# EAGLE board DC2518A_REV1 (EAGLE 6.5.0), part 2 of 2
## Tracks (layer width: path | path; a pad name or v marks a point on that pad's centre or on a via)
+2V5  (via drill 0.25)
  Top 0.152: v38.86,29.21 39.12,29.46 39.91,29.46 U9.13 U9.14
  Bottom 0.152: C41.1 v38.86,29.21
+3V3  (via drill 0.25)
  Top 0.152: U9.12 U9.11 38.59,30.5 v37.97,31.11 | v14.73,13.21 16.13,13.21 C15.1 16.22,13.21 17.02,13.21 17.45,12.78 U4.2 19.63,12.78 21.08,14.22 23.88,14.22 24.38,13.72 24.41,13.74 U3.6 | C50.1 84.07,18.76 84.07,19.56 84.29,19.77 U12.8 | 84.51,13.35 R80.R4_2 84.44,13.34 83.69,13.34 83.57,13.21 83.57,12.57 82.55,12.57 82.22,12.24 82.22,9.27 U11.18 | R66.2 v65.91,2.03 | SW1.SW1 15.29,29 15.62,29.46 25.27,29.46 v25.78,28.96 | R68.2 23.7,57.84 v24.38,57.28 | R69.2 53.34,56.9 53.85,56.39 v54.48,56.39 | v61.72,43.81 61.72,41.77 R58.2 | v69.09,45.97 69.48,46.37 R54.2 73.21,46.37 R53.2 C37.1
  Top 0.203: M10.2 94.68,35.21 C48.1 R72.1 R73.1 94.65,29.81 96.27,28.19 96.27,19.81 95.38,18.92 90,18.92 | R67.2 v22.99,2.03 | 90,19.43 90,18.92 | 90,18.92 R77.1 89.95,17.7 R81.1 | R80.R4_2 R80.R3_2 R80.R2_2 R80.R1_2 84.58,16.07 v84.58,17.02 84.58,17.27 84.16,17.69 C50.1 85.6,18.67 86.36,19.43 90,19.43 | v65.91,2.03 v77.22,2.03 | 90,19.43 90,20.45 R74.1 | R70.2 R71.1 25.95,29.12 v25.78,28.96
  Route2 0.152: v69.09,45.97 63.88,45.97 v61.72,43.81
  Route2 0.203: v14.73,2.03 v22.99,2.03 v44.45,2.03 v65.91,2.03 | v77.22,17.02 82.3,17.02 82.55,16.76 83.31,16.76 83.57,17.02 v84.58,17.02 | v37.97,31.11 v31.75,31.11 27.94,31.11 v25.78,28.96
  Route15 0.152: v54.48,56.39 58.04,56.39 61.72,52.7 v61.72,43.81 v61.72,32.38
  Route15 0.203: v14.73,2.03 v14.73,13.21 | v43.94,15.88 43.94,14.99 44.45,14.48 v44.45,2.03 | v77.22,2.03 v77.22,17.02 | v24.38,57.28 24.38,48.13 v31.75,40.01 v31.75,31.11 | v37.97,21.84 v37.97,31.11
  Bottom 0.152: 43.92,21.89 43.94,21.89 | 40.64,15.88 R16.1 | v25.78,28.96 25.78,27.9 R31.1 | C40.1 v37.97,31.11 | R36.2 31.24,40.51 v31.75,40.01 | R47.1 62.57,43.81 v61.72,43.81 | 42.56,22.35 R62.R1_2 42.61,21.84 v37.97,21.84 | 47.5,23.11 48.26,23.11 49.66,24.51 54.99,24.51 56.48,26 R65.2 R64.2 R63.2 56.48,32.38 58.93,32.38 | 47.5,23.11 46.99,23.11 45.85,21.89 R62.R4_2 | 58.93,32.38 v61.72,32.38 | v31.75,31.11 31.75,31.66 C45.1 30.48,32.51 28.96,32.51 28.32,33.15 U10.5 | 47.5,23.11 R14.1 47.79,22.19 47.88,22.1 49.02,22.1 49.66,21.59 50.29,21.59 50.55,21.34 M1.2 | R94.2 58.04,35.69 58.93,34.8 58.93,32.38
  Bottom 0.203: R62.R1_2 R62.R2_2 43.92,21.89 R62.R3_2 R62.R4_2 | 43.94,21.89 v43.94,15.88 40.64,15.88
+12V  (via drill 0.25)
  Top 0.152: 55.82,45.65 55.88,45.59 | 51.59,44.4 L2.1 | R93.2 R92.2 89.5,36.87 88.77,37.59 86.23,37.59 84.58,39.24 TP14.TP1
  Top 0.203: U7.3 55.82,45.65 | 55.88,45.59 55.88,44.7
  Top 0.229: 55.88,44.7 55.88,44.55 arc-90 55.73,44.4 55.63,44.4
  Top 0.254: 55.63,44.4 51.59,44.4
  Top 0.305: v48.26,45.72 v47.24,45.72 | v52.07,45.72 v52.96,45.72 v51.05,45.72 v50.16,45.72
  Bottom 0.305: C58.2 78.74,25.4 79.12,25.78 80.57,25.78 U14.20 80.64,29.59 81.53,30.48 81.92,30.48 81.92,31.53 U14.3
  other vias: 38.1,43.43 38.1,44.2 38.99,43.43 38.99,44.2
  pour Bottom (no thermals): 89.66,42.67 89.66,41.66 87.38,41.66 86.61,40.64 86.61,33.15 82.8,33.15 82.07,32.49 82.07,30.86 81.81,30.86 81.81,32.99 82.3,33.53 86.11,33.53 86.11,37.85 81.28,37.85 80.77,38.35 80.77,40.77 80.01,41.53 77.47,41.53 77.47,39.88 75.69,39.88 75.18,41.02 66.17,41.02 66.17,39.62 65.79,39.62 65.79,41.02 36.96,41.02 36.96,44.45 37.47,44.83 37.47,46.23 53.59,46.23 53.59,45.47 56.13,43.43 80.77,43.43 82.04,44.7 84.84,44.7 86.36,42.67
  pour Bottom (no thermals): 77.6,24.89 80.77,24.89 80.77,29.59 81.53,30.35 82.07,30.35 82.07,30.86 81.79,30.86 81.79,30.61 81.53,30.61 77.6,26.8
  pour Top (no thermals): 47.24,45.72 48.26,45.72 48.26,44.45 47.24,44.45
  pour Top (no thermals): 50.16,45.72 52.96,45.72 52.96,44.45 50.16,44.45
+12V_IN  (via drill 0.25)
  Top 0.152: v37.97,33.02 37.97,31.88 38.86,31 U9.10 | v98.04,43.18 98.72,42.51 R78.1 R83.2
  Route2 0.305: v92.71,39.12 89.15,35.56 v37.97,35.56
  Route15 0.305: v37.97,35.56 v37.97,33.02
  Route15 0.813: JP2.13 JP2.14
  Bottom 0.152: C39.1 v37.97,33.02 | v98.04,43.18 96.31,43.18 96.06,42.93
  Bottom 0.305: 93.98,42.16 93.98,39.12 v92.71,39.12
  Bottom 0.813: C52.2 96.01,45.09 96.01,48.47 J1.1 96.06,42.93 96.06,42.21 96.01,42.16 93.98,42.16 92.14,42.16 R84.I1
  pour Bottom (no thermals): 92.46,59.31 93.85,59.31 94.36,58.8 94.36,52.2 95.38,51.18 97.03,51.18 98.68,49.53 98.68,44.96 98.04,44.32 97.54,44.32 96.77,43.43 96.77,31.11 94.36,28.57 94.36,10.16 94.11,9.91 94.11,3.56 93.73,3.17 92.71,3.17 92.46,3.43 92.46,21.72 93.6,22.86 93.6,28.32 93.47,28.45 93.47,54.86 92.46,55.88
+15V  (via drill 0.25)
  other vias: 62.61,21.21 63.93,18.62 63.93,17.73 64.64,19.81
  pour Bottom (no thermals): 72.39,29.72 72.39,39.37 72.64,39.88 74.68,39.88 74.68,28.83 74.17,28.19 73.15,28.19 73.15,21.08 73.53,20.7 76.07,20.7 76.71,21.34 81.79,21.34 82.5,21.77 82.5,24.21 81.79,24.89 81.79,26.29 82.04,26.29 82.04,25.02 82.68,24.38 82.68,21.59 81.41,20.32 73.53,20.32 73.15,19.94 73.15,15.24 72.64,14.73 62.23,14.73 60.71,16.26 60.71,22.61 61.98,23.88 67.06,23.88
  pour Top (no thermals): 65.02,19.05 65.02,19.94 64.64,20.32 64.14,20.32 64.14,21.59 62.23,21.59 61.34,22.48 59.56,22.48 59.56,20.95 61.72,20.95 63.5,19.18 63.5,17.91 62.1,17.91 62.1,15.75 63.5,15.75 63.88,16.13 63.88,16.89 64.39,17.4 64.39,18.41
-15V  (via drill 0.25)
  Top 0.152: R19.2 26.38,12.41 26.67,12.7 28.07,12.7 28.07,13.46 | U3.1 25.91,16.99 25.91,15.7 | 28.07,15.7 U3.PAD
  Top 0.254: U4.4 18.09,11.12 18.16,11.05 v18.92,11.05
  Top 0.305: 25.91,15.7 28.07,15.7
  Top 0.406: U3.3 U3.2 U3.1 25.92,19.55 24.77,20.95 C11.1
  Route2 0.152: v89.15,18.49 88.9,18.29 v76.2,18.29
  Route15 0.152: v90.81,33.78 90.81,29.97 89.15,28.32 v89.15,18.49
  Bottom 0.152: R91.1 v89.15,18.49 | v76.2,18.29 76.17,18.32 D4.A
  Bottom 0.254: C14.1 v18.92,11.05
  other vias: 27.56,13.46 28.57,13.46 27.56,17.27 28.57,17.27
  pour Bottom (no thermals): 73.91,19.43 75.69,19.43 75.69,13.46 72.77,10.54 25.4,10.41 17.27,10.41 17.27,11.56 24,11.56 24,16 25.53,17.78 28.83,17.78 29.34,17.27 36.83,17.27 40.01,14.1 73.03,14.1 73.91,14.99 73.91,19.18 74.04,19.3
  pour Top (no thermals): 27.3,17.4 28.83,17.4 28.83,13.34 27.3,13.34
A0_MUX  (via drill 0.25)
  Top 0.152: U11.3 85.34,5.84 84.84,5.33 81.92,5.33 80.52,6.73 80.52,8.94 80.72,9.22 v80.7,9.65 80.7,10.03 80.52,10.21 80.52,10.67 80.64,10.79 80.64,14.48 81.28,15.11 82.57,15.11 R80.R2_1
  Bottom 0.152: JP3.6 81.79,8.64 80.77,9.65 v80.7,9.65
A1_MUX  (via drill 0.25)
  Top 0.152: U11.2 84.84,6.1 84.45,5.71 82.04,5.71 80.9,6.86 80.9,8.89 81.28,9.27 81.28,9.91 81.15,10.03 v81.15,10.41 81.15,10.79 81.03,10.92 81.03,11.43 81.15,11.56 81.15,13.84 81.66,14.35 82.57,14.35 R80.R3_1
  Bottom 0.152: JP3.7 81.79,9.91 81.28,10.41 v81.15,10.41
A2_MUX  (via drill 0.25)
  Top 0.152: U11.1 84.34,6.37 84.07,6.1 82.17,6.1 81.28,6.99 81.28,8.76 81.66,9.14 81.66,9.91 81.79,10.03 81.79,10.67 81.66,10.79 v81.66,11.18 81.66,13.34 81.79,13.46 82.57,13.46 R80.R4_1 82.49,13.34
  Bottom 0.152: JP3.8 v81.66,11.18
ALERTB  (via drill 0.25)
  Top 0.152: v47.75,24.13 47.75,25.78 47.88,25.91 47.88,26.16 | 47.88,26.16 47.88,26.42 47.7,26.59 U9.31 | v54.86,26.92 54.1,26.16 47.88,26.16
  Route2 0.152: v12.32,24.13 12.95,24.13 13.21,23.88 30.1,23.88 30.35,24.13 46.23,24.13 46.35,24.21 46.86,24.21 46.99,24.13 v47.75,24.13 | v54.86,26.92 v69.09,26.92 | v71.37,5.21 81.84,5.21 JP2.3 | v25.78,30.48 v12.32,30.48
  Route15 0.152: JP2.3 83.25,4.63 82.68,5.21 81.28,5.21 79.76,6.73 79.76,10.92 80.01,11.18 80.01,54.86 80.26,55.12 82.8,55.12 83.31,55.63 83.31,56.59 JP1.3 | v12.32,24.13 v12.32,30.48 12.32,33.53 TP10.TP | v69.09,26.92 69.09,7.49 v71.37,5.21
  Bottom 0.152: U10.1 28.97,31 28.45,30.48 v25.78,30.48 | R65.1 54.78,28.28 54.86,28.19 v54.86,26.92
CTRL  (via drill 0.25)
  Top 0.152: R82.2 90.68,30.99 92.71,28.96 S1.2 S1.5 92.71,20.61 C51.1 | U9.32 48.26,27.3 49.02,27.3 | U9.22 | U9.22 U9.23 | U9.33 49.02,27.93 49.02,27.3 | U9.22 43.2,26.57 42.93,26.29 v42.16,26.29 | 49.02,27.3 v49.91,27.3
  Route2 0.152: v49.91,27.3 54.36,27.3 54.61,27.56 68.71,27.56 69.09,27.94 v78.23,27.94 86.23,27.94 86.36,28.07 87.12,28.07 87.25,27.94 91.69,27.94 S1.2
  Route15 0.152: JP1.2 80.49,58.64 78.49,56.64 78.49,38.61 77.85,37.97 77.85,37.08 78.23,36.7 v78.23,27.94 78.23,5.84 80.01,4.06 80.01,3.03 JP2.2 | v42.16,26.29 42.16,25.78 42.93,25.02 43.69,25.02 44.2,25.53 44.2,26.04 45.47,27.3 v49.91,27.3
  Bottom 0.152: R64.1 53.59,30.86 53.59,27.3 v49.91,27.3
CTRL_P  (via drill 0.25)
  Top 0.152: R82.1 88.39,31.2 88.39,31.88 v89.03,32.51
  Route15 0.152: v89.03,32.51 89.28,32.77 TP8.TP
EESCL  (via drill 0.25)
  Route2 0.152: v102.5,12.97 102,12.97 101.35,12.32 v96.14,12.32
  Route15 0.152: J2.11 v102.5,12.97
  Bottom 0.152: R76.1 96.14,13.42 v96.14,12.32 95.25,12.32 95.25,10.54 96.27,9.78 96.27,8 95.57,7.56 U13.1
EESDA  (via drill 0.25)
  Route2 0.152: J2.12 104.5,21.83 99.57,16.89 96.39,16.89 v96.14,16.64
  Bottom 0.152: v96.14,16.64 96.14,15.53 R75.1 95.38,15.49 94.74,14.86 94.74,10.41 95.38,9.9 U13.3
FAULTB  (via drill 0.25)
  Top 0.152: 44.7,26.67 U9.25 U9.26 44.78,27.25 44.7,27.18 44.7,26.67 | 44.7,26.67 v44.7,25.27
  Route2 0.152: v13.21,25.4 24,25.4 24.51,24.89 29.84,24.89 30.1,25.15 43.18,25.15 43.31,25.02 43.81,25.02 44.07,25.27 v44.7,25.27 | v43.69,1.4 77.98,1.4 77.98,3.81 81.23,3.81 JP2.1 | v25.78,31.5 v13.21,31.5
  Route15 0.152: JP1.1 79.77,56.66 78.99,55.88 78.87,37.97 79.12,37.72 79.12,37.21 78.87,36.96 78.87,6.18 JP2.1 | TP9.TP 13.21,41.53 v13.21,31.5 v13.21,25.4 | v44.7,25.27 43.18,23.75 43.18,14.61 43.69,14.1 v43.69,1.4
  Bottom 0.152: U10.3 25.82,31.54 v25.78,31.5 | R62.R2_1 43.54,24.64 43.57,24.64 44.2,25.27 v44.7,25.27
GND  (via drill 0.25)
  Top 0.203: Q3.1 20.59,43.7 20.57,42.67 Q3.3
  other vias: 85.85,53.34 82.04,40.64 82.93,17.4 57.15,46.48 57.15,45.47 43.94,32.26 44.96,32.26 43.94,31.24 44.96,31.24
  pour Bottom (rank 2, no thermals): 0.51,0.51 0.51,62.99 106.17,62.99 106.17,0.51
  pour Top (rank 3): 0.51,0.51 106.17,0.51 106.17,62.99 0.51,62.99
  pour Route2 (no thermals): 0.51,0.51 106.17,0.51 106.17,62.99 0.51,62.99
  pour Route15 (no thermals): 0.51,0.51 106.17,0.51 106.17,62.99 0.51,62.99
  pour Route15: 86.61,55.63 86.87,55.63 86.87,53.85 86.36,53.34 86.36,50.29 86.87,49.78 86.87,44.7 86.61,44.45 86.61,43.94 86.87,43.69 86.87,16.51 86.61,16.26 86.36,16.51 86.36,21.59 86.61,21.84 86.61,22.35 86.36,22.61 85.34,22.61 85.09,22.23 85.09,21.72 85.34,21.34 85.34,12.7 86.11,11.94 86.11,7.11 85.34,6.35 83.31,6.35 82.55,7.11 82.55,8.64 82.8,8.89 82.8,12.7 81.53,13.97 81.53,24.64 82.8,24.64 82.8,23.88 85.6,23.88 85.85,24.13 85.85,24.64 85.34,25.15 84.58,25.15 84.07,25.65 81.53,25.65 81.53,46.74 85.09,50.29 85.09,53.59 86.36,54.86 86.61,54.86
  pour Top: 53.49,33.73 54.2,33.73 54.2,33.71 53.49,33.71
  pour Top: 52.76,34.11 52.78,34.11 52.78,33.45 52.76,33.45
  pour Bottom: 14.02,49.11 14.68,49.11 14.68,49.07 14.02,49.07
IIN_SNSM  (via drill 0.25)
  Top 0.152: v44.7,38.1 44.7,37.72 44.58,37.6 44.58,37.08 44.7,36.96 44.7,36.93 U9.56
  Route2 0.152: v88.65,39.12 87.76,38.23 55.24,38.23 54.99,37.97 52.96,37.97 52.83,38.1 v44.7,38.1
  Bottom 0.152: R84.E2 88.65,40.3 v88.65,39.12
IIN_SNSP  (via drill 0.25)
  Top 0.152: v45.21,37.34 45.2,37.33 U9.55 | U9.9 39.24,31.5 v38.86,31.88
  Route2 0.152: v91.44,39.12 91.44,38.73 88.65,36.07 65.79,36.07 65.02,36.78 64.26,36.78 64.14,36.7 49.28,36.7 49.15,36.78 48.9,36.78 48.77,36.7 45.85,36.7 v45.21,37.34 43.05,37.34 42.42,37.97 40.01,37.97 39.88,37.9 39.62,37.9 39.5,37.97 v38.86,37.97
  Route15 0.152: v38.86,31.88 v38.86,37.97
  Bottom 0.152: R84.E1 91.95,40.2 91.95,39.37 91.69,39.12 v91.44,39.12
ISNSN_CH0  (via drill 0.25)
  Top 0.152: U9.42 51.84,32.51 52.01,32.42 52.46,32.42 52.58,32.51 v53.85,32.51 U$40.P$2 | v72.01,8 R8.2 72.06,9.13 | R1.2 v68.33,15.88
  Route2 0.152: v54.61,8 v68.33,8 v72.01,8
  Route15 0.152: v53.85,32.51 53.85,9.02 v54.61,8 | v68.33,15.88 v68.33,8
ISNSN_CH1  (via drill 0.25)
  Top 0.152: v19.3,18.67 R20.2 21.46,18.76 | U9.44 48.95,33.53 49.53,33.53 49.66,33.45 50.16,33.45 50.29,33.53 v51.56,33.53 51.82,33.78 U$39.P$2 | R24.2 v19.3,9.14
  Route2 0.152: v51.56,19.05 47.24,19.05 46.99,19.3 19.94,19.3 v19.3,18.67
  Route15 0.152: v51.56,33.53 51.56,32.38 51.69,32.26 51.69,31.62 51.56,31.5 v51.56,19.05 | v19.3,9.14 19.3,10.41 19.56,10.67 19.56,11.43 19.3,11.68 v19.3,18.67
ISNSN_CH2  (via drill 0.25)
  Top 0.152: v51.05,34.54 50.29,34.54 50.16,34.67 49.66,34.67 49.53,34.54 48.99,34.54 U9.46
  Route2 0.152: v13.97,34.54 15.75,34.54 15.88,34.67 16.38,34.67 16.51,34.54 27.05,34.54 27.18,34.42 27.69,34.42 27.81,34.54 28.83,34.54 28.96,34.42 29.46,34.42 29.59,34.54 36.83,34.54 36.96,34.47 37.47,34.47 37.59,34.54 49.53,34.54 49.66,34.67 50.16,34.67 50.29,34.54 v51.05,34.54
  Route15 0.152: v14.48,43.81 13.97,43.31 v13.97,34.54
  Bottom 0.152: U$41.P$2 14.35,47.28 R39.2 14.39,45.01 C24.2 14.44,43.85 v14.48,43.81
ISNSN_CH3  (via drill 0.25)
  Top 0.152: U9.48 49.02,35.57 v49.02,36.2 | v72.39,43.56 72.77,43.56 72.9,43.69 R53.1 C37.2 76.33,44.87 TP30.1
  Route2 0.152: v49.02,36.2 v64.64,36.2 | v72.39,43.56 68.33,43.56 68.2,43.69 67.18,43.69 67.06,43.56 v65.79,43.56
  Route15 0.152: v64.64,36.2 65.79,37.34 v65.79,43.56
  Bottom 0.152: v65.79,43.56 M5.3
ISNSP_CH0  (via drill 0.25)
  Top 0.152: U9.41 49.65,32 49.78,32.08 50.04,32.08 50.16,32 50.93,32 v51.05,31.95 | v48.51,21.21 48.51,19.39 C7.1 R11.1 R12.1 48.3,14.48
  Route15 0.152: v51.05,31.95 51.05,27.18 48.77,24.89 48.77,21.59 v48.51,21.21 47.12,21.21 46.1,20.19 TP27.1
ISNSP_CH1  (via drill 0.25)
  Top 0.152: R25.1 R26.1 | U9.43 51.21,33.02 51.33,32.92 51.8,32.92 51.89,33.02 v52.2,33.02 | v41.91,16.64 41.4,16.64 41.02,16.26 R26.1 | C16.1 40.27,16.69 R26.1
  Route2 0.152: v51.56,16.64 v41.91,16.64
  Route15 0.152: v52.2,33.02 52.2,17.27 v51.56,16.64 | TP28.1 42.67,16 v41.91,16.64
ISNSP_CH2  (via drill 0.25)
  Top 0.152: v49.91,34.04 48.99,34.04 U9.45
  Route2 0.152: v16.13,34.04 27.05,34.04 27.18,33.91 27.69,33.91 27.81,34.04 28.83,34.04 28.96,33.91 29.46,33.91 29.59,34.04 v49.91,34.04 | TP29.1 16.13,54.86 v16.13,48.77
  Route15 0.152: v16.13,48.77 v16.13,34.04
  Bottom 0.152: U6.1 16.13,50.97 v16.13,48.77 16.13,47.28 R39.1 16.09,45.01 C24.1
ISNSP_CH3  (via drill 0.25)
  Top 0.152: U9.47 50.11,35 50.29,35.18 51.31,35.18 v51.94,34.54 | v70.36,44.2 R54.1
  Route2 0.152: v51.94,34.54 v70.61,34.54 | 72.14,44.2 v70.36,44.2
  Route15 0.152: v70.61,34.54 70.61,35.05 70.36,35.31 v70.36,44.2
N$1  (via drill 0.25)
  Top 0.152: v47.24,37.34 47.2,37.29 U9.51
  Bottom 0.152: v47.24,37.34 47.71,37.76 47.71,38.35 C43.1
N$2
  Top 0.152: R43.2 R42.1
N$3  (via drill 0.25)
  Top 0.152: v56.13,8.64 55.37,8.64 54.74,9.27 54.74,10.16 55.12,10.54 R6.1 | 62.48,18.5 U1.16 62.57,18.41 60.2,18.41 v60.2,19.3 | R5.2 53.12,18.2 53.34,18.41 57.04,18.41 U1.1 | R7.1 69.83,9.18 v70.61,9.17
  Top 0.203: v72.01,19.3 72.1,19.22 C6.1 72.1,16.42 72.39,16.13 72.39,15.28 U2.5
  Route2 0.152: v56.13,8.64 70.61,8.64 v70.61,9.17
  Route2 0.203: v72.01,19.3 64.9,19.3 64.77,19.18 64.01,19.18 63.88,19.3 v60.2,19.3
  Bottom 0.152: D7.A 59.69,18.8 v60.2,19.3
  pour Top (no thermals): 55.37,9.27 58.42,9.27 58.8,9.65 60.45,9.65 60.45,12.19 61.98,13.72 62.99,13.72 62.99,13.97 61.47,13.97 61.47,17.91 61.85,18.29 62.99,18.29 62.99,18.54 56.64,18.54 56.64,15.62 58.17,15.62 58.17,13.97 56.64,13.97 56.64,13.72 58.42,13.72 58.42,12.7 57.66,11.81 55.37,11.81
N$4
  Top 0.152: LED7.A 92.85,40.52 92.96,40.64 R83.1
N$5
  Top 0.152: U1.6 56.09,15.15 55.75,15.49 55.75,17.53 R5.1
N$6
  Top 0.152: U1.11 63.92,15.15 64.39,15.62 64.39,16.38 64.9,16.89 65.41,16.89 65.41,17.87 R2.1
N$7  (via drill 0.25)
  Top 0.152: R12.2 50.8,14.61 v51.18,14.48 | U1.10 62.61,14.48 v65.53,14.48 65.53,15.79 R1.1 65.41,15.84
  Route2 0.152: v51.18,14.48 v65.53,14.48
N$8  (via drill 0.25)
  Top 0.152: U2.4 72.52,13.27 72.52,12.45 73.53,11.43 73.53,6.73 61.59,6.73 TP3.TP | v54.74,12.19 54.74,10.92 54.36,10.54 R6.2 | R10.P$2 56.39,20.7 v56.39,19.81
  Route15 0.152: v56.39,19.81 54.74,18.54 v54.74,12.19
  pour Top (no thermals): 52.58,11.81 54.1,11.81 54.1,7.62 55.63,6.1 60.2,6.1 60.96,5.33 60.96,4.32 60.2,3.56 55.63,3.56 54.48,2.41 51.31,2.41 51.31,4.06 51.69,4.45 51.69,5.21 51.31,5.59 51.31,8 52.58,9.27
N$9
  Bottom 0.152: R38.1 17.4,50.2 17.4,52.83 16.15,52.83
  Bottom 0.203: 16.15,52.83 U6.3
N$10  (via drill 0.25)
  Top 0.152: U2.1 69.92,15.19 70.87,15.19 71.37,14.68 71.37,12.7 72.01,11.94 R8.1 71.34,10.92 v70.74,10.92 | R11.2 49.28,16.76 v49.28,10.29
  Route2 0.152: v49.28,10.29 70.36,10.29 v70.74,10.92
N$11
  Top 0.152: U3.8 29.21,14.39 29.21,18.54 29.84,19.05 30.73,19.05 | 30.73,19.05 30.7,19.81 R17.2 | C10.2 30.73,19.05
N$12  (via drill 0.25)
  Top 0.152: R18.2 34.04,19.81 34.04,21.55 R17.1 32.77,21.72 32,21.72 v30.99,22.86
  Bottom 0.152: v30.99,22.86 30.1,22.86 29.72,23.24 Q5.3
N$13  (via drill 0.25)
  Top 0.152: R21.1 v33.66,11.94 | v23.19,15.11 23.19,16.34 R22.1
  Route2 0.152: v33.66,11.94 v23.29,11.94
  Route15 0.152: v23.29,11.94 23.29,14.81 v23.19,15.11
  pour Top (no thermals): 33.66,17.27 29.72,17.27 29.72,15.62 31.62,15.62 32.38,14.86 32.38,12.57 34.92,12.57 34.92,13.84 33.66,15.11
N$14  (via drill 0.25)
  Route15 0.152: v30.99,18.54 29.46,17.02 29.46,9.14 v29.21,8.89
  Bottom 0.152: R28.2 30.99,19.3 v30.99,18.54 | v29.21,8.89 TP4.TP
  pour Top (no thermals): 29.97,12.06 29.97,6.86 29.21,6.1 28.83,6.1 27.94,5.21 27.94,4.32 28.7,3.56 32,3.56 32.77,2.79 35.69,2.79 35.69,5.71 35.43,5.97 35.43,8.38 34.92,8.89 34.92,11.05 30.73,11.05 30.73,12.06
N$15
  Top 0.152: U4.1 19.52,13.43 21.5,15.41 R22.2
N$16  (via drill 0.25)
  Top 0.152: R81.2 91.69,14.57 v91.69,13.59
  Bottom 0.152: v91.69,13.59 91.82,13.46 91.82,7.37 JP3.4
N$17  (via drill 0.25)
  Top 0.152: R26.2 37.47,16.26 v37.47,15.24 | U3.5 24.77,14.39 v24.77,15.24 24.77,17.78 24.13,18.54 23.24,18.54 23.24,18.63 R20.1
  Route2 0.152: v37.47,15.24 v24.77,15.24
N$18
  Top 0.152: U4.8 23.4,13.43 23.88,12.95 23.88,10.79 24.13,10.54 28.45,10.54 28.7,10.79 28.7,11.6 R23.2
N$19  (via drill 0.25)
  Top 0.152: R25.2 38.48,13.97 v38.48,10.16 | R24.1 22.06,9.99 22.35,10.29 | 22.35,10.29 22.35,11.42 U4.5 | 22.35,10.29 22.73,10.29 v23.11,10.16
  Route2 0.152: v38.48,10.16 v23.11,10.16
N$20
  Top 0.152: R35.2 R40.1 27.43,45.51 U5.3
  Top 0.203: R35.2 R34.1
N$21
  Bottom 0.152: Q5.2 30.67,29.72 24.13,29.72 24.13,27.81 R31.2 R32.2
N$22
  Top 0.254: U5.5 31.11,46.48 31.88,45.21 C20.1
N$23  (via drill 0.25)
  Top 0.152: C21.1 22.09,49.4 | v21.08,53.21 25.27,53.21 25.53,52.96 R37.1
  Bottom 0.152: R38.2 v21.08,53.21 | 18.67,50.99 18.67,51.82 21.08,51.82
  Bottom 0.203: U6.5 18.67,50.99 | 21.08,51.82 R38.2 C23.1
  pour Top (no thermals): 20.7,48.51 24.13,48.51 24.38,48.77 25.65,48.77 25.65,50.04 26.8,50.93 26.8,52.58 24.26,52.58 24.26,50.8 23.5,50.04 20.7,50.04
N$24  (via drill 0.25)
  Top 0.152: R50.2 71.48,52.25 71.48,52.76 71.27,52.93 69.55,52.93 69.47,52.91 69.34,52.83 R49.1 69.34,51.31 v71.37,51.31
  Bottom 0.152: v71.37,51.31 70.36,51.31 | 70.36,51.31 69.09,51.31 68.58,51.82 68.58,53.34 67.82,54.1 67.82,54.78 C35.2 | 70.36,49.4 70.36,48.51 69.98,48.16 69.22,48.16 68.58,48.77 U8.2 | 70.36,49.4 72.09,49.4 D5.A | 70.36,49.4 70.36,51.31
  pour Top (no thermals): 61.85,49.15 63.25,49.15 63.25,50.42 63.88,51.05 70.61,51.05 70.61,52.53 61.85,52.53
N$25
  Top 0.152: R66.1 64.1,5.8 63.88,5.59 LED1.A
N$26
  pour Top (no thermals): 26.8,47.12 28.07,47.12 28.07,48.01 28.57,48.51 28.83,48.51 29.46,49.15 29.46,50.04 30.48,50.8 30.48,53.98 29.08,53.98 29.08,51.31 27.69,49.91 27.69,48.77 26.8,48.13
N$27
  Top 0.152: U3.4 26.87,15.04 26.92,14.99 26.92,13.46 26.42,12.95 24.89,12.95 24.64,12.7 24.64,11.72 R19.1
N$28  (via drill 0.25)
  Top 0.152: R51.2 74.8,53.14 71.78,53.14 71.65,53.26 69.7,53.26 69.34,53.59 R49.2 | v66.78,50.34 66.64,50.13 R52.2 66.8,49.11 | v65.53,56.39 59.69,56.39 TP6.TP | R55.2 67.69,41.67 v67.69,42.6
  Route15 0.152: v65.53,56.39 65.53,51.56 v66.78,50.34 67.69,49.43 v67.69,42.6 67.69,37.34 67.06,36.7 v66.67,36.7
  Bottom 0.152: v66.67,36.7 66.29,36.21 R95.1
  pour Top (no thermals): 70.61,54.1 70.61,55.63 71.88,56.9 74.68,56.9 74.68,58.17 67.06,58.17 66.04,59.18 60.96,59.18 60.2,59.94 59.18,59.94 58.42,59.18 58.42,58.17 59.18,57.4 66.29,57.4 68.07,55.63 68.07,54.1
N$29  (via drill 0.25)
  Top 0.152: v37.85,53.47 40.64,53.47 40.77,53.43 R42.2 | R37.2 25.53,53.72 25.4,53.59 23.5,53.59 22.99,54.1 v20.19,54.1 | R34.2 21.59,41.06 v21.59,41.02
  Route2 0.152: v37.85,53.47 32.51,58.67 TP5.TP
  Route15 0.152: v21.59,41.02 20.19,41.02 v20.19,54.1
  Bottom 0.152: U6.4 20.13,52.89 20.19,52.96 v20.19,54.1
  pour Top (no thermals): 24.26,54.1 26.8,54.1 26.8,54.74 27.43,55.12 39.62,55.12 39.88,55.24 39.88,57.02 31.88,57.02 30.48,58.17 30.48,59.18 29.72,59.94 28.7,59.94 27.94,59.18 27.94,57.53 24.26,55.5
N$30  (via drill 0.25)
  Top 0.152: SW1.SW2 21.29,26.72 v22.99,24.77
  Route2 0.152: v22.99,24.77 23.5,24.77 23.88,24.38 29.97,24.38 30.23,24.64 46.99,24.64 47.12,24.77 56.01,24.77 56.39,25.15 v57.28,25.15
  Bottom 0.152: M2.1 59.69,23 59.69,23.5 59.09,24.09 R13.2 58.17,25.02 58.04,25.15 v57.28,25.15
N$31
  Top 0.152: U7.6 59.24,45.59 58.42,45.59 58.42,43.56 56.52,43.56 55.5,42.55 R45.1
N$32  (via drill 0.25)
  other vias: 34.29,47.12 35.05,47.12 35.05,47.88 34.29,47.88 34.29,48.64 35.05,48.64
  pour Top (no thermals): 29.46,47.62 29.46,47.12 31.24,47.12 31.75,46.61 35.43,46.61 35.43,54.1 31.5,54.1 31.5,50.8 33.78,50.8 33.78,48.13 31.62,48.13 31.11,47.62
  pour Bottom (no thermals): 37.08,45.72 37.08,46.99 35.69,48.26 35.69,49.28 33.78,49.28 33.78,46.74 34.8,45.72
N$33  (via drill 0.25)
  Top 0.152: v60.83,46.35 60.78,46.3 U7.7
  Bottom 0.152: C31.1 60.87,46.39 v60.83,46.35
N$34
  Bottom 0.152: R46.2 59.56,48.9 59.82,49.15 60.74,49.15 C32.1
N$35  (via drill 0.25)
  Top 0.152: U7.2 55.7,46.3 55.88,46.48 v55.88,48.77
  Bottom 0.152: R46.1 56.52,48.9 56.39,48.77 v55.88,48.77 55.63,48.51 55.63,44.45 C33.1
N$36  (via drill 0.25)
  Top 0.152: v54.99,47.62 U7.1 | R52.1 64.94,48.3 v64.9,48.26 | R59.1 57.26,42.56 v57.15,42.67
  Route2 0.152: v64.9,48.26 64.01,47.62 v54.99,47.62
  Route15 0.152: v57.15,42.67 56.01,42.67 54.99,43.69 v54.99,47.62
N$37  (via drill 0.25)
  Bottom 0.254: 51.44,49.02 v51.82,49.02 51.82,49.53 51.05,49.53 v51.05,49.02 51.44,49.02 | 51.44,49.02 C29.2
  pour Top (no thermals): 55.37,45.09 55.37,44.83 54.23,44.83 53.98,45.09 53.98,46.23 53.47,46.74 49.78,46.74 49.78,49.28 52.83,50.04 54.1,51.31 55.12,51.31 55.12,49.66 54.23,48.77 54.23,45.21 54.36,45.09
N$38  (via drill 0.25)
  Top 0.152: LED1.C v63.25,3.17
  Bottom 0.152: v63.25,3.17 67.56,3.17 M6.3
N$39  (via drill 0.25)
  Top 0.254: v55.75,54.23 56.52,54.23 56.77,53.98 56.77,53.08 D2.A
  Bottom 0.254: R48.1 55.71,54.14 v55.75,54.23
  pour Top (no thermals): 56.13,49.78 57.78,49.78 58.42,49.15 60.07,49.15 60.07,52.58 57.53,52.58 57.53,53.47 56.13,53.47
N$40
  Top 0.152: R67.1 24.8,5.8 25.02,5.59 LED2.A
N$41  (via drill 0.25)
  Top 0.152: v25.65,3.17 LED2.C
  Bottom 0.152: M7.3 21.34,3.17 v25.65,3.17
N$42
  pour Bottom (no thermals): 80.77,30.99 80.01,30.99 78.99,32.38 77.98,33.66 76.07,33.66 76.07,35.56 85.72,35.56 85.72,33.91 81.92,33.91 80.77,32.77
N$43
  Top 0.152: R68.1 23.88,59.42 LED3.A
N$44  (via drill 0.25)
  Top 0.152: v83.82,30.48 83.82,31.24 82.55,32.51 82.55,33.4 v78.49,37.47
  Bottom 0.152: R85.1 R86.2 78.45,37.63 v78.49,37.47 | v83.82,30.48 83.82,31.62 U14.6
N$45  (via drill 0.25)
  Top 0.152: LED3.C 25.65,58.67 20.45,58.67 v20.45,57.71
  Bottom 0.152: v20.45,57.71 20.45,57.73 M8.3
N$46
  Bottom 0.152: C57.1 84.45,22.35 83.89,22.92 U14.15
N$47
  Bottom 0.152: U14.8 85.19,30.76 85.34,30.61 87.38,30.61 87.88,31.11 88.56,31.11 C56.1
N$48
  Bottom 0.152: U14.7 84.54,30.77 84.99,30.3 90.75,30.3 90.93,30.48 R87.2
N$49
  Top 0.152: R69.1 54.36,59.42 LED4.A
N$50
  pour Bottom (no thermals): 81.15,26.42 81.41,26.42 81.41,24.64 82.17,23.88 82.17,22.1 81.66,21.72 76.45,21.72 75.95,21.21 73.91,21.21 73.91,23.5 80.26,23.5 81.15,24.51
N$51
  Top 0.152: R78.2 100.42,39.37 | 100.42,39.37 R79.1 | M10.1 94.68,39.05 95,39.37 100.42,39.37
N$52
  Bottom 0.152: U14.16 83.24,26.6 83.44,26.8 87.12,26.8 88.01,25.91 88.01,21.21 | 88.01,21.21 86.91,21.21 R90.1 | R91.2 89.11,21.21 88.01,21.21
N$53  (via drill 0.25)
  Top 0.152: v49.91,31.5 U9.40
  Bottom 0.152: C44.1 49.57,31.84 v49.91,31.5
N$55  (via drill 0.25)
  Route2 0.152: v76.71,29.46 81.66,29.46 v82.68,30.48
  Bottom 0.152: R89.2 75.65,28.36 75.56,28.45 75.56,29.43 | 75.56,29.43 R88.1 | 75.56,29.43 76.67,29.43 v76.71,29.46 | v82.68,30.48 83.06,30.48 83.19,30.61 83.19,31.5 U14.5
N$56
  Bottom 0.406: C29.1 52.7,53.09 52.83,52.07 R48.2
N$57  (via drill 0.25)
  Top 0.152: R51.1 v74.8,49.78
  Bottom 0.152: 67.57,49.66 U8.3 67.63,48.7 68.58,47.75 70.36,47.75 70.74,48.13 73.15,48.13 v74.8,49.78
N$58  (via drill 0.25)
  Top 0.152: LED4.C 56.13,58.67 50.93,58.67 v50.93,57.71
  Bottom 0.152: v50.93,57.71 50.93,57.73 M9.3
N$60
  Bottom 0.152: R61.2 72.22,52.67 D5.C | 69.59,52.45 U8.5 69.53,53.79 69.47,53.85 69.47,54.83 C35.1
  Bottom 0.203: U8.5 69.71,52.58 72.14,52.58 D5.C
N$61  (via drill 0.25)
  Top 0.152: R50.1 v72.39,55.12
  Route15 0.152: v64.52,50.42 v64.52,53.21
  Bottom 0.152: v72.39,55.12 71.63,55.88 66.8,55.88 66.8,54.1 67.56,53.34 67.56,52.46 U8.4 67.57,52.45 66.8,52.45 66.04,53.21 v64.52,53.21 | M5.2 66.55,47.19 66.55,48.01 65.53,49.02 C36.1 64.52,49.95 v64.52,50.42
N$62
  Bottom 0.152: U8.1 69.53,50.61 69.27,50.88 67.13,50.88 66.45,51.56 65.62,51.56 C36.2 64.73,51.65 63.88,50.8 63.88,47.14 64.77,47.14 M5.1
N$63  (via drill 0.25)
  Top 0.152: U1.7 56.16,14.5 55.63,13.97 R3.1 54.74,13.93 54.61,13.46 54.61,13.21 53.59,12.45 C5.1 50.04,12.53 v50.04,13.46
  Route15 0.152: v51.56,17.78 51.05,17.78 50.04,16.76 v50.04,13.46
  Bottom 0.152: 53.59,18.93 D7.C | M1.6 52.22,23.01 52.32,23.11 52.32,23.5 52.58,23.75 53.85,23.75 54.36,23.24 54.36,19.94 53.85,19.56 53.85,18.92 D7.C | D7.C 52.58,18.8 v51.56,17.78
N$64
  Top 0.152: LED5.A R70.1
N$65
  Top 0.152: LED6.A R71.2
N$66  (via drill 0.25)
  Top 0.152: R77.2 88.14,17.74 88.14,16.64 87.88,16.38 C49.1 | U11.4 85.84,6.1 v85.98,5.97 | v86.61,15.37 87.8,15.37
  Top 0.203: 87.8,15.37 C49.1
  Route15 0.152: v85.98,5.97 86.61,6.6 v86.61,15.37
N$67  (via drill 0.25)
  Top 0.152: LED6.C v27.43,35.05
  Bottom 0.152: v27.43,35.05 27.69,34.8 27.69,33.76 U10.4
N$68  (via drill 0.25)
  Top 0.152: LED5.C v29.21,35.05
  Bottom 0.152: v29.21,35.05 28.96,34.8 28.96,33.76 U10.6
N$70
  Top 0.152: R7.2 69.47,11.94 69.98,12.45 69.98,13.24 U2.3
N$71
  Bottom 0.152: M1.4 49.55,22.34 49.78,22.1 50.93,22.1 51.56,21.46 51.56,20.7 M1.1 53.34,20.68 R15.1
N$72
  Bottom 0.152: M4.3 37.34,47.5 37.59,47.24 38.5,47.24 M3.1 38.63,47.24 39.5,47.24 39.84,47.59 R33.1
N$73  (via drill 0.25)
  Top 0.152: v54.36,38.61 54.1,38.35 54.1,37.1 LED10.A
  Bottom 0.152: R94.1 54.78,38.19 v54.36,38.61
N$74  (via drill 0.25)
  Top 0.152: U12.1 84.29,23.54 v85.79,22.04 87.25,20.57 R74.2 | U11.9 86.88,9.77 86.74,9.91 86.74,10.79 86.87,10.92 86.87,12.45 86.61,12.7 86.23,12.7 v85.98,12.95
  Route15 0.152: v85.98,12.95 85.98,13.46 85.85,13.59 85.85,21.59 v85.79,22.04
N$75
  Bottom 0.152: U15.4 65.79,37.38 65.79,36.96 65.28,36.45 65.28,34.54 65.55,34.27 R95.2 R96.2 C62.2
N$77  (via drill 0.25)
  Top 0.152: R55.1 R56.2 64.66,39.51 v64.64,39.5
  Bottom 0.152: v64.64,39.5 61.17,39.5 C61.1 61.03,39.33 59.11,39.33 R97.1
PG_+15V  (via drill 0.25)
  Top 0.152: LED8.A R92.1 87.88,35.85 v87.88,34.8
  Route2 0.152: v83.82,32.64 84.84,32.64 87,34.8 v87.88,34.8
  Bottom 0.152: U14.4 82.59,32.3 82.93,32.64 v83.82,32.64
PG_-15V  (via drill 0.25)
  Top 0.152: LED9.A 86.87,33.78 | 86.87,33.78 R93.1 | v86.87,33.02 86.87,33.78
  Route15 0.152: v86.74,27.43 86.74,32.89 v86.87,33.02
  Bottom 0.152: U14.17 82.59,26.71 83.06,27.18 86.36,27.18 v86.74,27.43
REFP  (via drill 0.25)
  Top 0.152: v49.91,30.48 48.97,30.48 U9.38 | v62.74,40.39 62.74,41.62 R56.1 | R57.1 69.45,40.4 v69.47,40.39
  Route2 0.152: v69.47,40.39 v62.74,40.39 v50.49,40.39 | v33.91,30.48 v49.91,30.48
  Route15 0.152: v49.91,30.48 50.49,30.48 v50.49,40.39
  Bottom 0.152: C44.2 49.57,30.14 v49.91,30.48 | R29.1 R30.1 33.87,30.48 v33.91,30.48
RESETB  (via drill 0.25)
  Top 0.152: SW2.SW1 16.89,36.07 v16.89,36.96 | U9.24 44.2,26.54 43.94,26.16 v43.56,25.65
  Route2 0.152: v43.56,25.65 29.97,25.65 29.59,25.27 25.4,25.27 24.77,25.91 17.27,25.91 v16.89,26.04 | v87.25,44.2 75.31,44.2 74.04,42.93 68.33,42.93 67.94,43.31 67.44,43.31 67.06,42.93 57.91,42.93 57.4,43.43 v43.18,43.43
  Route15 0.152: JP2.7 87.25,27.05 87.38,27.18 87.38,27.69 87.25,27.81 87.25,32.38 87.5,32.64 87.5,33.4 87.25,33.66 v87.25,44.2 87.25,50.04 86.87,50.42 86.87,53.34 87.25,53.72 JP1.7 | v16.89,26.04 v16.89,36.96 | v43.18,43.43 43.18,28.32 43.56,27.94 v43.56,25.65
  Bottom 0.152: R62.R1_1 42.67,25.13 43.18,25.65 v43.56,25.65 | v16.89,36.96 16.3,36.96 C42.1
RUN_CH0  (via drill 0.25)
  Top 0.152: U9.3 39.29,34.5 39.24,34.54 39.24,36.45 38.35,37.34 36.96,37.34 36.83,37.41 36.32,37.41 36.2,37.34 v35.81,37.34
  Route2 0.152: v35.81,18.67 v46.74,18.67 46.99,18.41 57.53,18.41 59.69,20.57 TP15.1 | v66.55,7.37 v47.24,7.37
  Route15 0.152: v35.81,37.34 v35.81,18.67 | v47.24,7.37 47.24,17.27 46.74,17.78 v46.74,18.67
  Bottom 0.152: M6.1 66.9,6.96 v66.55,7.37 | v46.74,18.67 47.5,19.43 R14.2 47.84,20.49 47.88,20.45 48.51,20.45 48.75,20.69 M1.3
RUN_CH1  (via drill 0.25)
  Top 0.152: U3.7 30.22,13.01 v30.23,12.98 | U9.4 39.28,34 38.86,34.42 38.86,36.32 38.35,36.83 v36.58,36.83
  Route2 0.152: v30.23,8.89 30.23,7.62 v20.7,7.62 | v30.23,12.98 30.35,13.08 36.45,13.08 38.48,15.11 v38.48,17.78
  Route15 0.152: v30.23,12.98 v30.23,8.89 | v36.58,36.83 36.58,19.68 v38.48,17.78 | TP20.1 17.27,9.78 19.43,7.62 v20.7,7.62
  Bottom 0.152: v20.7,7.62 20.7,6.17 M7.1 | R16.2 39.46,17.61 39.37,17.65 39.12,17.78 v38.48,17.78
RUN_CH2  (via drill 0.25)
  Top 0.152: U9.5 39.95,33.53 39.24,33.53 38.48,34.29 38.48,35.18 38.53,35.31 38.53,35.81 37.97,36.32 36.96,36.32 36.83,36.25 36.32,36.25 36.2,36.32 v35.18,36.32 | U5.4 29.98,44.8 v29.97,44.2
  Route2 0.152: v19.56,59.69 19.56,43.94 29.54,43.94 v29.97,44.2
  Route15 0.152: v36.32,49.02 36.32,42.67 35.18,42.67 | v35.18,36.32 35.18,42.67 | 35.18,42.67 31.33,42.67 30.02,43.83 v29.97,44.2 | TP23.1 17.53,58.67 18.54,59.69 v19.56,59.69
  Bottom 0.152: v19.56,59.69 20.64,59.69 M8.1 | M4.1 36.69,49.52 v36.32,49.02 | R36.1 30.27,43.78 v29.97,44.2
RUN_CH3  (via drill 0.25)
  Top 0.152: U7.5 v59.3,44.2 v59.31,44.2 | U9.6 38.86,33 38.86,33.4 v37.21,35.05
  Route2 0.152: v37.21,40.77 41.02,40.77 42.42,42.16 42.42,44.2 v59.31,44.2 | TP26.1 46.35,57.02 48.64,59.31 v50.04,59.31
  Route15 0.152: v37.21,35.05 v37.21,40.77 | v50.04,59.31 50.04,56.9 52.2,54.74 54.3,54.74 58.17,50.88 58.17,45.34 v59.31,44.2
  Bottom 0.152: v59.31,44.2 59.31,44.32 59.94,44.96 R47.2 | M9.1 50.35,59.62 v50.04,59.31
SCL  (via drill 0.25)
  Top 0.152: v47.24,26.16 47.24,27.21 U9.30 | U12.2 83.64,24.71 v83.31,24.38
  Route2 0.152: TP12.TP 19.05,27.3 19.43,27.69 25.4,27.69 25.65,27.94 27.43,27.94 27.69,27.69 45.72,27.69 v47.24,26.16 74.17,26.16 75.18,25.15 82.55,25.15 v83.31,24.38
  Bottom 0.152: v47.24,26.16 47.24,25.02 45.59,25.02 45.24,24.66 R62.R4_1
SCL_IN  (via drill 0.25)
  Top 0.152: R73.2 97.28,30.99 v98.3,30.1 103.41,30.1 J2.4 | U11.19 81.92,8.77 v81.92,8 | U12.3 82.99,27.49 83.19,27.69 84.71,27.69 85.22,27.18 v85.22,24.38
  Route2 0.152: v85.22,24.38 89.03,24.38 89.53,24.89 98.3,24.89 v98.3,30.1
  Route15 0.152: JP1.6 86.23,57.67 86.23,55.5 84.58,53.85 84.58,50.55 81.03,46.99 81.03,25.15 | 81.03,25.15 81.03,13.59 82.22,12.39 82.22,9.07 81.92,8.76 v81.92,8 81.92,6.86 82.8,5.97 84.96,5.97 86.23,4.7 86.23,2.54 85.49,1.79 JP2.6 | v85.22,24.38 84.58,24.38 83.82,25.15 81.03,25.15
SDA  (via drill 0.25)
  Top 0.152: U9.29 46.61,27.16 v46.61,23.62 | v83.31,22.99 83.64,22.66 U12.7
  Route2 0.152: TP13.TP 9.65,20.57 12.45,23.37 30.1,23.37 30.35,23.62 41.15,23.62 v41.53,23.24 42.04,23.62 v46.61,23.62 47.37,23.62 47.5,23.55 48.01,23.55 48.13,23.62 52.45,23.62 52.58,23.75 57.15,23.75 57.61,24.21 58.42,24.21 58.55,24.38 69.34,24.38 69.47,24.21 69.98,24.21 70.1,24.13 82.17,24.13 v83.31,22.99
  Bottom 0.152: R62.R3_1 44.32,24.2 44.32,22.86 42.29,22.86 41.91,23.24 v41.53,23.24
SDA_IN  (via drill 0.25)
  Top 0.152: R72.2 97.54,33.02 v98.93,31.75 101.6,31.75 101.85,32 103.44,32 J2.2 | U11.20 84.07,8.27 84.07,7.87 86.74,7.87 86.74,5.71 85.98,4.95 84.71,4.95 84.25,4.5 84.25,2.72 83.45,1.92 JP2.4 | U12.6 82.99,20.52 v83.06,20.45
  Route2 0.152: v83.06,20.45 v98.93,20.45 | v98.93,5.84 87.5,5.84 86.23,4.57 86.23,3.3 85.72,2.79 84.25,2.79 JP2.4
  Route15 0.152: JP1.4 83.04,58.66 82.3,57.91 82.3,55.63 80.01,55.63 79.5,55.12 79.5,11.43 79.38,11.3 79.38,6.48 81.03,4.83 82.3,4.83 82.3,2.75 JP2.4 | v98.93,31.75 v98.93,20.45 v98.93,5.84
SHARE_CLK  (via drill 0.25)
  Top 0.152: JP1.5 85.25,55.28 84.58,54.61 82.55,54.61 82.3,54.36 82.3,51.94 TP7.TP | U9.18 41.2,25.96 40.64,25.4 v40.64,22.86
  Route2 0.152: v40.64,22.86 40.89,22.61 56.9,22.61 v57.91,23.62 66.29,23.62 66.42,23.75 67.18,23.75 67.31,23.62 v69.72,23.62 | v71.37,6.1 82.95,6.1 JP2.5
  Route15 0.152: JP2.5 85.25,4.92 84.58,5.59 81.66,5.59 80.14,7.11 80.14,10.67 80.52,11.05 80.52,50.42 TP7.TP | v57.91,23.62 v57.91,33.53 | v69.72,23.62 69.72,7.75 v71.37,6.1
  Bottom 0.152: JP3.5 83.01,6.04 83.13,5.91 JP2.5 | v57.91,33.53 57.91,34.54 54.86,34.54 54.86,33.4 R63.1
TSENSE_CH0  (via drill 0.25)
  Top 0.152: U9.15 38.91,28.5 v38.61,28.25 | v65.79,9.65 65.79,8.87 Q1.2 66.39,8.85 66.67,9.14 67.42,9.14 C9.1
  Route2 0.152: v39.88,9.65 v65.79,9.65
  Route15 0.152: v38.61,28.25 38.61,18.92 39.88,17.65 v39.88,9.65
TSENSE_CH1  (via drill 0.25)
  Top 0.152: Q2.2 28.99,21.72 28.83,21.84 28.83,22.86 C18.1 28.83,22.88 v28.83,25.91 | v39.88,26.29 39.95,26.36 U9.16
  Route2 0.152: v28.83,25.91 29.21,26.29 v39.88,26.29
TSENSE_CH2  (via drill 0.25)
  Top 0.152: v18.41,45.97 19.28,45.21 Q3.2 | U9.27 45.7,26.4 v45.59,26.04
  Route2 0.152: v45.59,26.04 44.96,26.04 44.07,26.92 27.43,26.92 27.05,27.3 26.04,27.3 25.65,26.92 v20.19,26.92
  Route15 0.152: v20.19,26.92 20.19,27.94 18.41,29.72 v18.41,43.94
  Bottom 0.152: v18.41,45.97 18.41,44.96 | 18.41,44.96 v18.41,43.94 | C26.1 18.41,44.96
TSENSE_CH3  (via drill 0.25)
  Top 0.152: Q4.2 62.66,44.96 63.5,44.96 | U9.34 48.95,28.45 v49.91,28.45 | v63.5,43.81 63.5,44.96 | 63.5,44.96 64.17,44.96 C38.1
  Route2 0.152: v49.91,28.45 v63.5,28.45
  Route15 0.152: v63.5,28.45 v63.5,43.81
UNUSED1
  Route15 0.152: JP1.9 89.25,55.5 90.17,55.5 91.57,54.1 91.57,50.8 89.79,49.02 89.79,30.23 87.76,28.19 87.76,6.22 89.28,4.83 89.28,3.83 JP2.9
UNUSED2
  Route15 0.152: JP2.10 90.27,2.84 90.27,4.83 88.27,6.73 88.27,28.07 90.17,29.97 90.17,48.77 92.08,50.67 92.08,54.23 90.3,56.01 90.3,57.66 89.3,58.66 JP1.10
USB_3.3V  (via drill 0.25)
  Top 0.152: v99.95,34.8 99.95,34.92 98.04,36.83 97.03,36.83 96.52,37.34 96.52,37.78 M10.3
  Route15 0.152: v99.95,34.8 99.95,30.23 101.35,30.23 102.47,29.07 J2.5
USB_5V
  pour Bottom (no thermals): 103.38,33.91 103.38,32.26 101.6,32.26 101.09,31.75 101.09,12.7 100.33,11.94 100.33,7.87 95.12,2.67 88.65,2.67 88.14,2.29 88.14,1.02 86.61,1.02 86.61,2.92 92.46,2.92 92.58,2.84 93.85,2.84 93.98,2.92 94.74,2.92 99.19,7.37 99.19,9.27 97.41,9.27 97.41,15.88 99.57,15.88 99.57,17.53 100.33,18.8 100.46,32.89 101.6,33.91
  pour Top (no thermals): 101.85,32.51 103.25,32.51 103.25,34.42 105.41,36.45 105.41,52.2 97.16,60.45 87.12,60.45 86.44,59.69 86.44,57.91 88.06,57.91 88.06,59.18 88.77,59.82 96.77,59.82 104.78,51.82 104.78,36.7 102.49,34.42 101.85,34.42
VDAC_CH0  (via drill 0.25)
  Top 0.152: R3.2 R4.1 v52.15,15.75 | U9.53 46.2,37.18 v46.35,37.34
  Route2 0.152: v46.61,39.62 46.99,39.37 v52.07,39.37 | v68.33,16.89 66.93,16.89 65.79,15.75 v52.15,15.75
  Route15 0.152: v46.35,37.34 46.35,39.37 v46.61,39.62 | v52.07,39.37 52.07,38.23 52.83,37.72 52.83,24.38 52.58,24.13 52.58,16.64 52.15,16.2 v52.15,15.75 | TP16.1 68.33,21.59 v68.33,16.89
VDAC_CH1  (via drill 0.25)
  Top 0.152: U9.54 45.72,36.27 45.72,36.96 45.8,37.08 45.8,37.59 45.72,37.72 v45.72,40.01
  Route2 0.152: v45.72,40.01 33.15,40.01 32.38,40.77 27.05,40.77 26.54,40.26 v26.54,40.01
  Route15 0.152: v26.54,40.01 v26.54,26.67 26.54,25.65 22.99,22.1 TP18.1
  Bottom 0.152: v26.54,26.67 26.16,26.67 25.91,26.42 25.91,24.8 R32.1
VDAC_CH2  (via drill 0.25)
  Top 0.152: R40.2 v27.43,40.01 | v44.2,39.24 44.2,39.37 44.2,38.48 44.07,38.35 44.07,37.85 44.2,37.72 U9.57
  Route2 0.152: v27.43,40.01 28.19,39.24 29.72,39.24 | 29.72,39.24 v44.2,39.24 | TP21.1 29.72,39.24
VDAC_CH3  (via drill 0.25)
  Top 0.152: R58.1 R59.2 58.55,41.66 58.55,40.64 51.31,40.64 50.93,41.02 v45.21,41.02 43.7,41.02 43.7,39.64 43.61,39.5 43.61,38.99 43.69,38.86 U9.58
  Route15 0.152: TP24.1 45.21,53.59 v45.21,41.02
VSNSM_CH1  (via drill 0.25)
  Top 0.152: U9.64 40.7,37.02 40.39,37.34 40.39,39.12 38.61,39.12 38.1,38.61 v34.54,38.61
  Route15 0.152: v34.54,38.61 34.54,24.13 v33.27,22.86 31.24,20.83 TP19.1
  Bottom 0.152: R29.2 32.17,20.66 32.51,20.32 33.53,20.32 33.87,19.98 R28.1 | v33.27,22.86 33.27,22.61 33.02,22.35 33.02,21.59 R29.2 | C17.1 R29.2
VSNSM_CH3  (via drill 0.25)
  Top 0.152: U9.50 47.7,36.83 47.83,36.96 47.83,37.62 48.51,38.35 v48.51,40.01
  Route2 0.152: v48.51,40.01 49.15,40.01 49.4,39.75 51.44,39.75 51.69,40.01 52.58,40.01 53.21,39.37 v56.64,39.37
  Route15 0.152: v48.51,40.01 45.72,42.8 45.72,52.83 TP25.1
  Bottom 0.152: R97.2 v56.64,39.37 56.39,39.62 R98.1
VSNSP_CH0  (via drill 0.25)
  Top 0.152: v56.39,21.46 56.39,22.21 R10.P$3 R10.P$4 53.16,22.21 | U9.1 39.88,35.57 39.88,36.07 39.75,36.2 v39.75,38.48 | C8.1 52.22,22.21 53.09,22.21 53.16,22.21 | v53.16,23.16 53.16,22.21
  Route2 0.152: v39.75,38.48 40.01,38.61 44.45,38.61 44.58,38.68 44.83,38.68 44.96,38.61 v53.34,38.61 | TP17.1 56.77,21.84 v56.39,21.46
  Route15 0.152: v53.34,38.61 53.34,32.89 53.21,32.77 53.21,32.26 53.34,32.13 53.34,24 53.16,23.82 v53.16,23.16
  Bottom 0.152: v56.39,21.46 56.9,21.97 M2.3
VSNSP_CH1  (via drill 0.25)
  Top 0.152: U9.63 41.2,37.34 v41.15,37.34
  Route2 0.152: v41.15,37.34 36.83,37.34 36.32,37.97 35.31,37.97 35.18,37.85 v32.51,37.85
  Route15 0.152: v32.51,37.85 32.51,23.11 v32.26,22.86
  Bottom 0.152: v32.26,22.86 32.26,23.79 R30.2
VSNSP_CH2  (via drill 0.25)
  Top 0.152: U9.61 42.16,36.25 42.19,36.35 42.19,37.19 v42.04,37.34 | v42.04,46.99 41.15,46.99 | R43.1 41.15,46.99 | 41.15,46.99 R44.2
  Route2 0.152: TP22.1 17.53,41.91 19.56,39.88 25.15,39.88 26.92,41.66 v36.07,41.66
  Route15 0.152: v42.04,37.34 42.04,41.66 | 42.04,41.66 v42.04,46.99 | v36.07,41.66 42.04,41.66
  Bottom 0.203: C25.1 42.71,47.66 v42.04,46.99
VSNSP_CH3  (via drill 0.25)
  Top 0.152: U9.49 48.2,37.05 v48.39,37.34 | v70.99,37.34 70.99,39.5 70.74,39.75 70.74,41.64 R57.2
  Route2 0.152: v48.39,37.34 v70.99,37.34
  Route15 0.152: TP31.1 46.35,43.18 49.15,40.39 49.15,38.1 v48.39,37.34
  Bottom 0.152: 68.31,35.69 R96.1 | U15.1 67.75,39.43 67.44,39.12 67.44,37.21 67.94,36.7 R96.1 | 68.18,35.56 R96.1 | v70.99,37.34 70.99,36.32 70.36,35.69 69.71,35.69 C62.1 R96.1

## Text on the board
tPlace: INSTALL CONNECTORS | +48V | -48V | ON TOP SIDE | RUN2 | ISP2 | F | E | M | A | L | E | RUN3 | GND | VSP2 | 0.1A | 0.1A | 9-14V | VDAC3 | VSM3 | - | + | VSP3 | ISN3 | SHARE_CLK | CTRL | VDAC2 | +12V | FAULT | CH2 | CH3 | VDD33 | +15V | FAULT | ALERT | LTC2975 | -15V | ALERT | RESET | DEMO CIRCUIT 2518A | High | Voltage | & | Negative | Voltage | Power | System | Management | FAULT | RUN | OFF | SCL | VDAC0 | VDAC1 | VSM1 | CH1 | CH0 | VSP0 | RUN1 | RUN0 | SDA | ISP1 | ISP0 | 0.25A | 0.25A | GND | M | A | L | E | GND | -12V | +12V
bPlace: Rev 1 | mtp | LTC CONFIDENTIAL | FOR CUSTOMER USE ONLY | A2 | A1 | A0 | SCLK | OPEN
tStop: LTC2975CUP | 4-CHANNEL POWER | SYSTEM MANAGER | (408) 432-1900 | www.linear.com
bStop: SYSTEM MANAGER | 4-CHANNEL POWER | LTC2975CUP | (408) 432-1900 | www.linear.com
d_TopPastemask: NOTES: UNLESS OTHERWISE SPECIFIED | 1. COPPER PADS WITH 2 MIL SPACING ARE INTENTIONALLY | DESIGNED AS SUCH (PASTE MASK OPENING INTENDED | TO SHORT PADS TOGETHER) | COPPER PADS HAVE INTENTIONAL 2 MIL SPACING
d_BotPastemask: NOTES: UNLESS OTHERWISE SPECIFIED | 1. COPPER PADS WITH 2 MIL SPACING ARE INTENTIONALLY | DESIGNED AS SUCH (PASTE MASK OPENING INTENDED | TO SHORT PADS TOGETHER) | PADS HAVE INTENTIONAL 2 MIL SPACING
d_FabDrawing: 2.50" | BOTTOM PADS HAVE INTENTIONAL 2 MIL SPACING | TOP PADS HAVE INTENTIONAL 2 MIL SPACING | 0.00" | 0.00" | 4.20"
